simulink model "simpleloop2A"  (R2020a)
settings: Solver=ode45  StartTime=0.0  StopTime=10.0  RelTol=1e-3  EnableMultiTasking=on

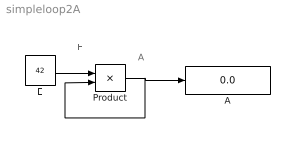
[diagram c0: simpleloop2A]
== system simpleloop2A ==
  note: A
  note: E
  note: .
  A : Display
  E : Constant  Value=42
  Product : Product  Inputs=*/  SaturateOnIntegerOverflow=on
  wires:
  E/1 -> Product/1
  Product/1 -> A/1, Product/2
